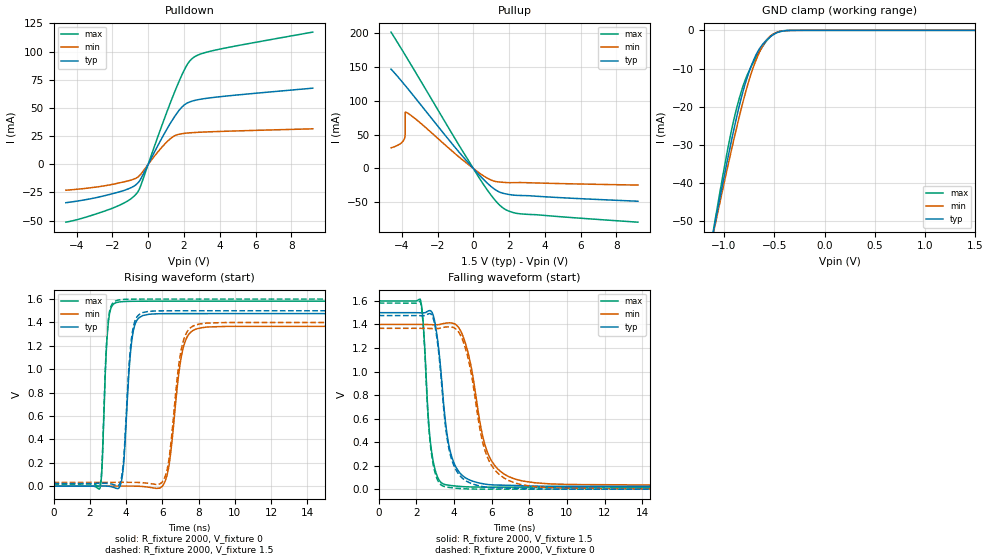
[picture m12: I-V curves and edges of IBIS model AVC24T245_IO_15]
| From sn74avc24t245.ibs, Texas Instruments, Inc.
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[Model]   AVC24T245_IO_15
Model_type  I/O
Vinl=0.49
Vinh=1.04
Enable   Active-Low
Vref =   0
Rref =   2000
Cref =   15p
Vmeas =   0.75
| variable   typ   min   max
C_comp   5.18pF   4.55pF   5.77pF
| C_pullup   5.10pF   3.65pF   7.53pF
| C_pulldown   4.79pF   4.27pF   5.46pF
| C_tri-state   5.18pF   4.55pF   5.77pF
[Temperature Range]   40   100   -40
| Ambient temperature   25   85   -40
[Voltage range]   1.5   1.4   1.6
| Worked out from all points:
|   slope of the pulldown table from 0 to 0.225 V, typ, clamps not added: 32.1 ohm
|   slope of the pullup table from 0 to 0.225 V, typ, clamps not added: 33.9 ohm
|   GND clamp passes 1 mA (typ) near -0.50 V on its own axis
|   rising waveform, R_fixture 2000, V_fixture 0: 20-80 % time 355ps typ, 581ps min, 237ps max; typ from 0 V to 1.48 V
|   falling waveform, R_fixture 2000, V_fixture 1.5: 20-80 % time 628ps typ, 1ns min, 383ps max; typ from 1.5 V to 0.023 V
|   rising waveform, R_fixture 2000, V_fixture 1.5: 20-80 % time 351ps typ, 568ps min, 235ps max; typ from 0.023 V to 1.5 V
|   falling waveform, R_fixture 2000, V_fixture 0: 20-80 % time 629ps typ, 997ps min, 376ps max; typ from 1.48 V to 0 V
[GND Clamp]
| AVC24T245_IO_15
|   Voltage   I(typ)   I(min)   I(max)
-4.6V     -597.8mA   -546.6mA   -662.5mA
-1.1V     -52.11mA   -52.52mA   -51.59mA
-1.075V   -48.66mA   -49.4mA    -47.7mA
-930mV    -29.5mA    -31.88mA   -26.82mA
-830mV    -17.94mA   -20.74mA   -16.24mA
-765mV    -12.02mA   -14.35mA   -11.48mA
-685mV    -6.644mA   -8.056mA   -7.261mA
-605mV    -3.35mA    -3.664mA   -3.806mA
-535mV    -1.602mA   -1.422mA   -1.608mA
-460mV    -500.6uA   -413.1uA   -383.6uA
-350mV    -38.76uA   -40.58uA   -15.38uA
1.5V      804.6pA    34.44nA    79.67pA
[Pulldown]
| AVC24T245_IO_15
|   Voltage   I(typ)   I(min)   I(max)
-4.6V     -34.07mA   -23.01mA   -51.35mA
-1.885V   -25.62mA   -17.44mA   -38.24mA
-1.09V    -21.68mA   -14.59mA   -31.97mA
-630mV    -17.39mA   -11.88mA   -25.55mA
-415mV    -12.94mA   -8.777mA   -18.95mA
595mV     18.22mA    11.97mA    26.91mA
1.265V    37.01mA    23.01mA    55.56mA
1.7V      47.29mA    26.56mA    72.61mA
2.03V     52.78mA    27.45mA    84.03mA
2.5V      56.24mA    28.09mA    94.31mA
3.84V     59.63mA    29.04mA    101.6mA
9.2V      67.51mA    31.46mA    117.2mA
[Pullup]
| AVC24T245_IO_15
|   Voltage   I(typ)   I(min)   I(max)
-4.6V     146.8mA    30.47mA    201.5mA
-4.1V     131.8mA    36.24mA    180.2mA
-3.85V    123.9mA    43.96mA    169.4mA
-3.81V    122.6mA    49.37mA    167.6mA
-3.805V   122.5mA    83.3mA     167.4mA
-3.785V   121.8mA    83.17mA    166.5mA
-3.155V   101.3mA    71.56mA    138.8mA
175mV     -5.197mA   -3.574mA   -7.497mA
980mV     -26.35mA   -16.94mA   -39.04mA
1.625V    -36.35mA   -20.39mA   -57.65mA
2.595V    -39.89mA   -20.78mA   -66.9mA
9.2V      -48.41mA   -24.54mA   -79.36mA
[Ramp]
| AVC24T245_IO_15
| variable   typ   min   max
dV/dt_r   0.90/3.68E-10   0.83/5.92E-10   0.96/2.49E-10
dV/dt_f   0.90/6.38E-10   0.83/1.01E-09   0.96/3.92E-10
R_load = 2000
[Rising Waveform]
| AVC24T245_IO_15
R_fixture =   2000
C_fixture =   0
L_fixture =   0
V_fixture =   0
V_fixture_min = 0
V_fixture_max = 0
|   Time   V(typ)   V(min)   V(max)
0s        19.4nV     97.73nV    508.8pV
2.56ns    903.7uV    -145.4uV   -16.02mV
2.99ns    17.08uV    136.1uV    1.348V
3.425ns   -16.9mV    569.1uV    1.568V
4.36ns    1.291V     545.2uV    1.581V
4.925ns   1.459V     -2.673mV   1.582V
6.19ns    1.475V     56.87mV    1.582V
7.08ns    1.475V     1.134V     1.582V
7.865ns   1.475V     1.344V     1.582V
29.99ns   1.476V     1.367V     1.582V
[Falling Waveform]
| AVC24T245_IO_15
R_fixture =   2000
C_fixture =   0
L_fixture =   0
V_fixture =   1.5
V_fixture_min = 1.4
V_fixture_max = 1.6
|   Time   V(typ)   V(min)   V(max)
0s        1.5V       1.4V       1.6V
2.205ns   1.499V     1.4V       1.616V
2.795ns   1.511V     1.398V     339.2mV
3.115ns   1.288V     1.398V     108.3mV
3.475ns   685mV      1.409V     41.66mV
3.805ns   319.5mV    1.413V     31.8mV
4.35ns    131.5mV    1.347V     22.94mV
5.74ns    40.93mV    330.1mV    17.41mV
7.215ns   31.29mV    87.55mV    17.21mV
29.99ns   23.49mV    32.46mV    17.19mV
[Rising Waveform]
| AVC24T245_IO_15
R_fixture =   2000
C_fixture =   0
L_fixture =   0
V_fixture =   1.5
V_fixture_min = 1.4
V_fixture_max = 1.6
|   Time   V(typ)   V(min)   V(max)
0s        23.49mV    32.45mV    17.19mV
2.56ns    24.39mV    32.33mV    1.842mV
2.995ns   23.35mV    32.62mV    1.382V
3.485ns   3.954mV    33.1mV     1.588V
4.33ns    1.298V     32.85mV    1.599V
4.91ns    1.484V     29.77mV    1.6V
6.175ns   1.5V       91.41mV    1.6V
7.04ns    1.5V       1.165V     1.6V
7.81ns    1.5V       1.377V     1.6V
29.99ns   1.5V       1.4V       1.6V
[Falling Waveform]
| AVC24T245_IO_15
R_fixture =   2000
C_fixture =   0
L_fixture =   0
V_fixture =   0
V_fixture_min = 0
V_fixture_max = 0
|   Time   V(typ)   V(min)   V(max)
0s        1.476V     1.367V     1.582V
2.205ns   1.474V     1.367V     1.597V
2.79ns    1.486V     1.365V     319.2mV
3.105ns   1.271V     1.365V     86.71mV
3.45ns    691.1mV    1.375V     24.57mV
3.785ns   306.3mV    1.379V     14.13mV
4.32ns    113.6mV    1.317V     5.422mV
5.715ns   16.97mV    296.8mV    207.5uV
7.21ns    7.307mV    54.88mV    21.64uV
29.99ns   70.94nV    3.562uV    60.54nV
